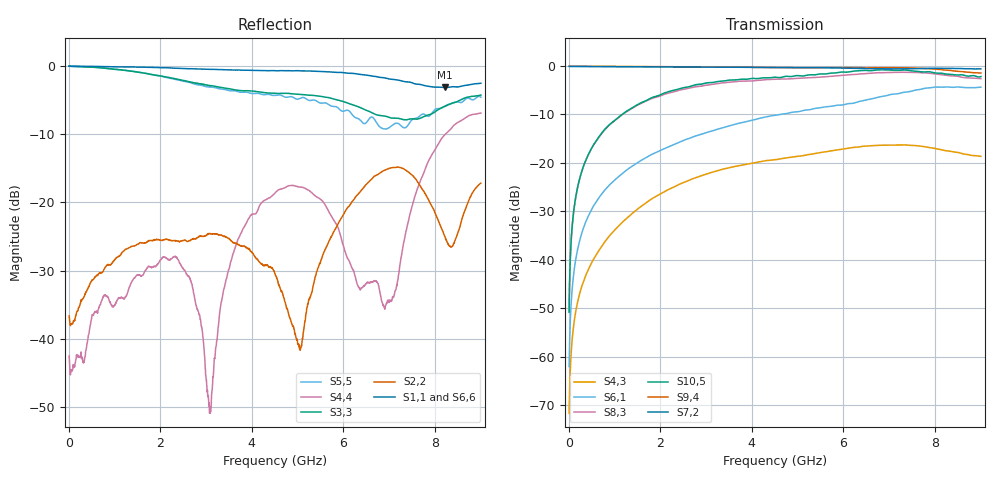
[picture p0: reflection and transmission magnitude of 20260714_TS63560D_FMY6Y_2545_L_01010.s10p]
# GHz S DB R 50
! CMT, SN0916, 25263762, 26.7.0
! Date: 15.07.2026 13:38:29
! Data: Format
! Freq S1.1:dB/Ang S1.2:dB/Ang S1.3:dB/Ang S1.4:dB/Ang S1.5:dB/Ang S1.6:dB/Ang S1.7:dB/Ang S1.8:dB/Ang S1.9:dB/Ang S1.10:dB/Ang
!  S2.1:dB/Ang S2.2:dB/Ang S2.3:dB/Ang S2.4:dB/Ang S2.5:dB/Ang S2.6:dB/Ang S2.7:dB/Ang S2.8:dB/Ang S2.9:dB/Ang S2.10:dB/Ang
!  S3.1:dB/Ang S3.2:dB/Ang S3.3:dB/Ang S3.4:dB/Ang S3.5:dB/Ang S3.6:dB/Ang S3.7:dB/Ang S3.8:dB/Ang S3.9:dB/Ang S3.10:dB/Ang
!  S4.1:dB/Ang S4.2:dB/Ang S4.3:dB/Ang S4.4:dB/Ang S4.5:dB/Ang S4.6:dB/Ang S4.7:dB/Ang S4.8:dB/Ang S4.9:dB/Ang S4.10:dB/Ang
!  S5.1:dB/Ang S5.2:dB/Ang S5.3:dB/Ang S5.4:dB/Ang S5.5:dB/Ang S5.6:dB/Ang S5.7:dB/Ang S5.8:dB/Ang S5.9:dB/Ang S5.10:dB/Ang
!  S6.1:dB/Ang S6.2:dB/Ang S6.3:dB/Ang S6.4:dB/Ang S6.5:dB/Ang S6.6:dB/Ang S6.7:dB/Ang S6.8:dB/Ang S6.9:dB/Ang S6.10:dB/Ang
!  S7.1:dB/Ang S7.2:dB/Ang S7.3:dB/Ang S7.4:dB/Ang S7.5:dB/Ang S7.6:dB/Ang S7.7:dB/Ang S7.8:dB/Ang S7.9:dB/Ang S7.10:dB/Ang
!  S8.1:dB/Ang S8.2:dB/Ang S8.3:dB/Ang S8.4:dB/Ang S8.5:dB/Ang S8.6:dB/Ang S8.7:dB/Ang S8.8:dB/Ang S8.9:dB/Ang S8.10:dB/Ang
!  S9.1:dB/Ang S9.2:dB/Ang S9.3:dB/Ang S9.4:dB/Ang S9.5:dB/Ang S9.6:dB/Ang S9.7:dB/Ang S9.8:dB/Ang S9.9:dB/Ang S9.10:dB/Ang
!  S10.1:dB/Ang S10.2:dB/Ang S10.3:dB/Ang S10.4:dB/Ang S10.5:dB/Ang S10.6:dB/Ang S10.7:dB/Ang S10.8:dB/Ang S10.9:dB/Ang S10.10:dB/Ang
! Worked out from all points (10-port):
!   2001 points, 10 MHz to 9 GHz, reference 50 ohm
!   strongest paths, dB at 10 MHz, 2.257 GHz, 4.505 GHz, 6.753 GHz, 9 GHz:
!     S7,2: -0.1, -0.2, -0.3, -0.6, -0.6
!     S9,4: -0.1, -0.2, -0.4, -0.4, -1.5
!     S10,5: -50.7, -5.1, -2.4, -0.8, -2.2
!     S8,3: -50.7, -5.5, -2.8, -1.4, -2.6
!     S6,1: -62.0, -16.4, -10.2, -6.5, -4.4
!     S4,3: -71.6, -25.2, -19.3, -16.4, -18.7
!   lowest |S11| = -3.1 dB at 8.222 GHz (marker M1), VSWR 5.60, Z = 11 - j23.7 ohm
!   |S11| at or under -10 dB: nowhere
